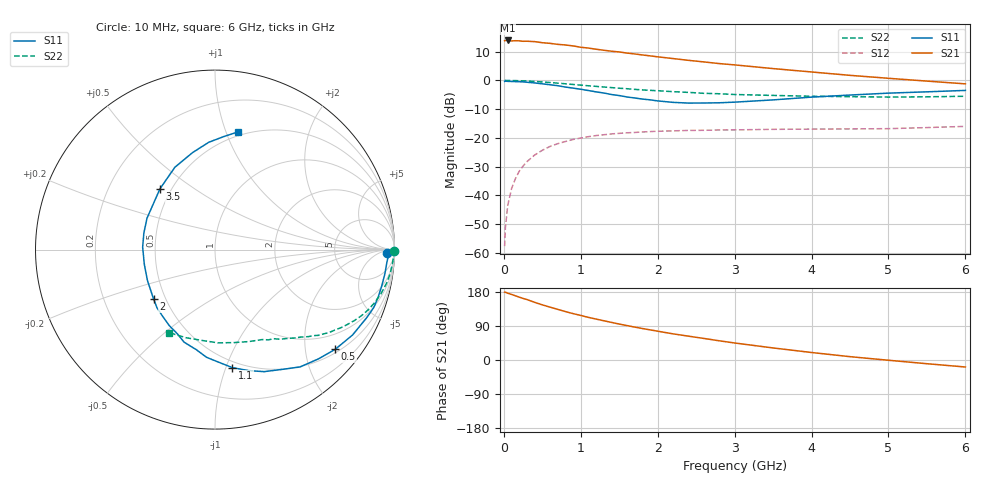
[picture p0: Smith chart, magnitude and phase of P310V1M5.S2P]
! SIEMENS Small Signal Semiconductors
! BFP181
! Si NPN RF Bipolar Junction Transistor in SOT143
! VCE = 10 V  IC = 1.5 mA
! Common Emitter S-Parameters:  March  1996
# GHz  S  MA  R  50
!  f  S11  S21  S12  S22
! GHz  MAG  ANG  MAG  ANG  MAG  ANG  MAG  ANG
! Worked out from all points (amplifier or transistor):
!   36 points, 10 MHz to 6 GHz, reference 50 ohm
!   highest |S21| = 13.9 dB at 50 MHz (marker M1)
!   |S21| within 3 dB of that: start of sweep to 1.186 GHz
!   unconditionally stable (mu >= 1): 2.88 GHz to end of sweep
!   at 250 MHz: K = 0.11, MSG = 21.7 dB, |S12| = -29.8 dB
!   at 1.4 GHz: K = 0.55, MSG = 14.4 dB, |S12| = -18.7 dB
!   at 6 GHz: K = 1.20, MAG = 4.7 dB, |S12| = -16.0 dB
!   S11 on the Smith chart (normalised r, x): 10 MHz: 40, -17; 500 MHz: 0.58, -2.66; 1.1 GHz: 0.45, -1.05; 2 GHz: 0.43, -0.29; 3.5 GHz: 0.43, +0.37; 6 GHz: 0.47, +1.10
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0.01  0.9586 -1.0  4.905 179.1  0.0013 79.6  0.9958 -0.3
0.02  0.9682 -1.7  4.943 178.9  0.0027 86.9  0.9953 -0.8
0.05  0.9609 -3.9  4.947 176.4  0.0066 87.6  0.9945 -2.0
0.1  0.9561 -8.1  4.851 173.1  0.013 84.4  0.993 -3.8
0.2  0.9469 -16.2  4.868 165.9  0.0262 79.7  0.985 -7.7
0.3  0.9272 -24.0  4.796 159.6  0.0384 74.4  0.9731 -11.3
0.4  0.9022 -31.8  4.723 152.2  0.0501 69.9  0.9569 -14.9
0.5  0.8702 -39.7  4.519 145.5  0.0606 65.1  0.9377 -18.3
0.6  0.8382 -46.6  4.405 139.6  0.0707 60.6  0.9177 -21.4
0.8  0.7637 -61.0  4.13 127.8  0.0862 52.6  0.8712 -27.0
0.9  0.7329 -68.1  3.974 122.4  0.0936 48.7  0.8471 -29.5
1.1  0.6648 -81.6  3.646 112.4  0.1047 42.4  0.8039 -33.9
1.3  0.6019 -94.5  3.339 103.5  0.1131 37.2  0.766 -37.8
1.5  0.544 -108.4  3.12 94.8  0.1195 32.7  0.7292 -41.1
1.8  0.4726 -128.1  2.768 83.1  0.1262 27.4  0.6822 -45.6
2  0.4388 -141.3  2.567 76.0  0.1301 24.2  0.6597 -48.3
2.2  0.4138 -155.5  2.394 69.0  0.1321 21.5  0.6351 -51.3
2.8  0.407 166.8  1.959 50.7  0.137 15.1  0.5843 -59.4
3.5  0.457 132.1  1.602 31.8  0.1404 10.4  0.5465 -69.6
4.5  0.5548 103.0  1.222 8.8  0.1427 5.7  0.52 -88.1
5.5  0.6315 85.6  0.97 -9.8  0.1506 5.5  0.517 -108.4
6  0.6683 78.9  0.869 -18.5  0.1581 4.4  0.5286 -119.0
